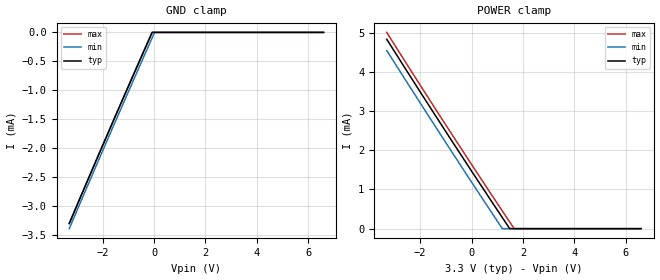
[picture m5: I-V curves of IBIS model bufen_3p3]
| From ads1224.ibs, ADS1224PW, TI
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|   bufen_3p3 Model
[Model]   bufen_3p3
Model_type   Input
Vinl = 0.66
Vinh = 2.64
|   typ   min   max
|   (nom PVT)   (fast PVT)   (slow PVT)
|C_comp from frequency sweep method (F= 8MHz)
|Average
C_comp   8.705e-16   7.366e-16   1.045e-15
|C_comp from LC tank measurement(L=1nH)
|Average
|Resonant Frequency(Hz)   1.000e+12   1.000e+12   1.000e+12
|C_comp   2.536e-17   2.536e-17   2.536e-17
[Model spec]
Vinl   0.66   0.6   0.72
Vinh   2.64   2.4   2.88
| Where nom  PVT is Nominal Process, 3.3V, 25C
|   Fast PVT is Strong Process,  3.6V, -40C
|   Slow PVT is Weak Process,   3V, 85C
[Voltage Range]   3.3   3   3.6
|Ambient Temperature   25   85   -40
|Junction Temperature
[Temperature Range]   25   85   -40
[Power Clamp Reference]   3.3   3   3.6
[GND Clamp Reference]   0   0   0
[GND Clamp]
|   Voltage   I(typ)   I(min)   I(max)
-3.3V     -3.298mA   -3.386mA   -3.297mA
-1.759V   -1.707mA   -1.798mA   -1.701mA
-78mV     -7.485uA   -99.41uA   -244.9nA
21mV      0A         0A         0A
6.6V      0A         0A         0A
[POWER Clamp]
|   Voltage   I(typ)   I(min)   I(max)
-3.3V     4.834mA    4.548mA    5.009mA
-1.136V   2.615mA    2.334mA    2.784mA
1.2V      282.3uA    394.9nA    452.6uA
1.485V    2.055uA    0A         173.2uA
1.661V    0A         0A         1.144uA
6.6V      0A         0A         0A
